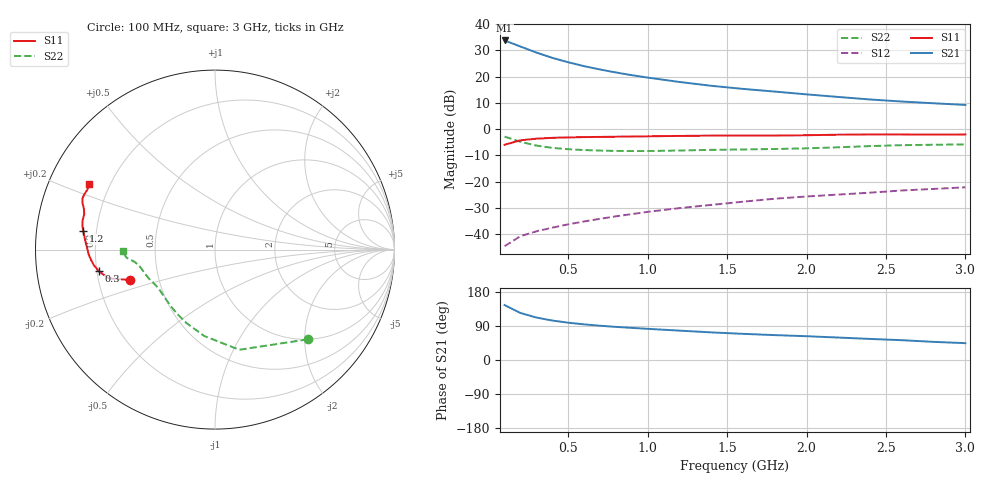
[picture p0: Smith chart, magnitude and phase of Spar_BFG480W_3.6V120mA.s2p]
! Filename: 3_6120BFG480.001
! Title: BFG480W
! Bias: Vce=3.6V; Ic=120mA
! Company: NXP Semiconductors NL
! User: Quality&Reliability T&D
! Measure time: 10 Nov 1999 / 12:01:24
#  MHz  S  MA  R 50
! Freq  S11  S21  S12  S22  :
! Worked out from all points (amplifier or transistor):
!   20 points, 100 MHz to 3 GHz, reference 50 ohm
!   highest |S21| = 33.8 dB at 100 MHz (marker M1)
!   |S21| within 3 dB of that: start of sweep to 229.4 MHz
!   unconditionally stable (mu >= 1): 619.4 MHz to end of sweep
!   at 400 MHz: K = 0.87, MSG = 32.4 dB, |S12| = -37.6 dB
!   at 1.2 GHz: K = 1.09, MAG = 22.2 dB, |S12| = -30.1 dB
!   at 3 GHz: K = 1.06, MAG = 14.2 dB, |S12| = -22.2 dB
!   S11 on the Smith chart (normalised r, x): 100 MHz: 0.34, -0.15; 300 MHz: 0.21, -0.09; 1.2 GHz: 0.15, +0.07; 3 GHz: 0.12, +0.24
100  0.5036 -160.4  49.09 145.0  0.005863 68.5  0.7189 -44.1
200  0.6122 -164.8  37.57 124.0  0.009107 61.3  0.5742 -76.4
300  0.6579 -169.4  28.83 112.1  0.01125 61.2  0.4853 -97.0
400  0.6821 -172.9  22.87 104.2  0.01321 63.2  0.4391 -111.1
500  0.6951 -175.7  18.83 98.5  0.01529 65.5  0.4141 -121.1
600  0.7051 -178.0  15.89 94.0  0.01734 67.5  0.3992 -128.5
700  0.7105 180.0  13.73 90.5  0.01947 69.4  0.3897 -134.1
800  0.7162 178.1  12.04 87.4  0.02172 71.0  0.3841 -138.8
900  0.7235 176.3  10.7 84.8  0.02395 72.6  0.3819 -142.9
1000  0.7297 174.7  9.615 82.2  0.02646 73.5  0.3826 -146.5
1200  0.7418 171.9  7.932 77.5  0.03115 74.9  0.3912 -152.3
1400  0.7514 169.7  6.709 72.9  0.03589 75.6  0.4023 -156.5
1600  0.7554 167.4  5.851 69.1  0.04133 76.1  0.4094 -159.8
1800  0.7548 164.8  5.201 65.7  0.04709 76.5  0.4179 -163.4
2000  0.7652 162.7  4.603 62.8  0.05194 77.1  0.4301 -167.5
2200  0.7826 160.6  4.106 59.3  0.05647 76.8  0.4504 -171.0
2400  0.7919 158.9  3.677 55.6  0.06144 76.2  0.4748 -173.3
2600  0.7906 157.2  3.361 52.3  0.06764 75.4  0.4941 -174.7
2800  0.7856 154.9  3.114 47.9  0.07238 74.0  0.5038 -176.5
3000  0.7903 152.2  2.891 44.4  0.07779 73.1  0.5119 -179.3
